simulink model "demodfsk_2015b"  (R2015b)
settings: Solver=VariableStepAuto  SolverMode=SingleTasking  StartTime=0.0  StopTime=10.0  RelTol=1e-3
libraries: simulink x1, commfilt2 x1, dspsrcs4 x1

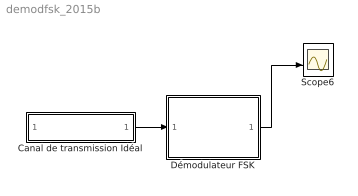
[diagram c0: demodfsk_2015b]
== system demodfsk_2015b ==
  Canal de transmission Idéal : Subsystem
  Démodulateur FSK : Subsystem
  Scope6 : Scope  NumInputPorts=2
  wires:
  Canal de transmission Idéal/1(Out1) -> Démodulateur FSK/1(In1)
  ? -> Scope6/1
  Démodulateur FSK/1(Out1) -> Scope6/2
  ? -> Canal de transmission Idéal/1(In1)

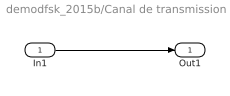
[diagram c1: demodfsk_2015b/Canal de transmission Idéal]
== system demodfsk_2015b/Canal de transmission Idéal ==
  In1 : Inport
  Out1 : Outport
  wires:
  In1/1 -> Out1/1

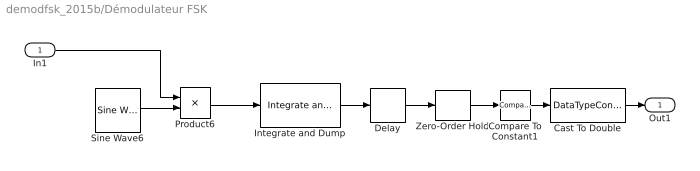
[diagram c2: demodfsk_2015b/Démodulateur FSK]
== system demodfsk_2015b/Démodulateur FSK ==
  In1 : Inport
  Cast To Double : DataTypeConversion  OutDataTypeStr=double
  Compare To Constant1 : simulink/Logic and Bit Operations/Compare To Constant  relop=>  const=0.5  OutDataTypeStr=boolean
  Delay : Delay  DelayLength=1
  Integrate and Dump : commfilt2/Integrate and Dump  obssamples=100  offsetsamples=0  nodump=on  roundingMode=Floor  overflowMode=off
  Product6 : Product
  Sine Wave6 : dspsrcs4/Sine Wave  Amplitude=1  Frequency=1  Phase=0  SampleMode=Discrete  OutComplex=Real  CompMethod=Trigonometric fcn  TableSize=Speed  SampleTime=1/100  SamplesPerFrame=1  ResetState=Restart at time zero  OutputFrames=off  dataType=double  wordLen=16  udDataType=sfix(16)  fracBitsMode=Best precision  numFracBits=15  OutDataTypeStr=double  LastOutDataTypeStr=double
  Zero-Order Hold : ZeroOrderHold
  Out1 : Outport
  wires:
  Integrate and Dump/1 -> Delay/1
  Sine Wave6/1 -> Product6/2
  In1/1 -> Product6/1
  Product6/1 -> Integrate and Dump/1
  Delay/1 -> Zero-Order Hold/1
  Zero-Order Hold/1 -> Compare To Constant1/1
  Cast To Double/1 -> Out1/1
  Compare To Constant1/1 -> Cast To Double/1
